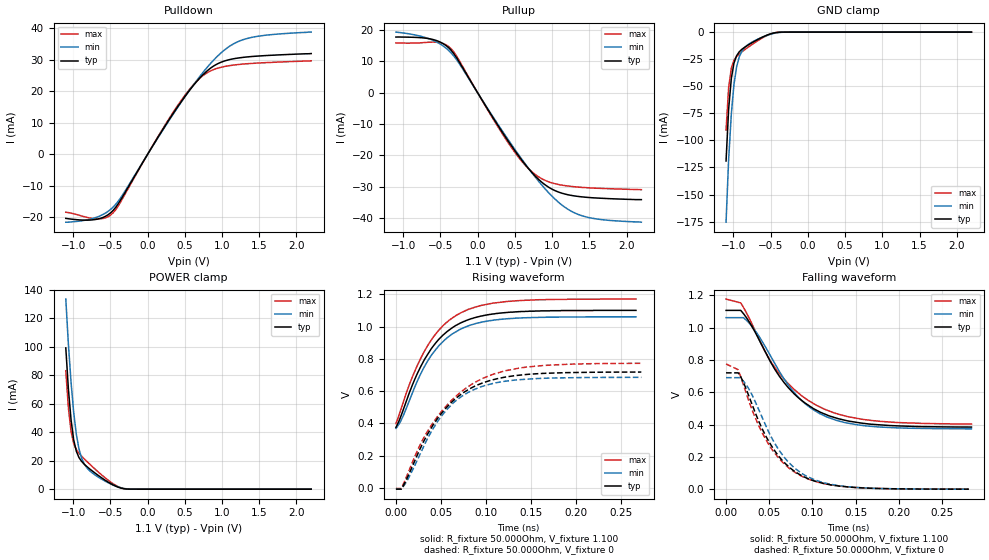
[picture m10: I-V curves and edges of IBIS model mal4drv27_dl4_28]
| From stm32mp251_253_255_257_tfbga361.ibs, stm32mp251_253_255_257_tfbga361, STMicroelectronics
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[Model] mal4drv27_dl4_28
Model_type   I/O
Polarity   Non-Inverting
Enable   Active-High
C_comp   1.656pF   1.654pF   1.662pF
C_comp_pullup   832.475fF   825.290fF   839.619fF
C_comp_pulldown 737.556fF   736.745fF   750.731fF
Vinh = 413.000mV
Vinl = 293.000mV
Vmeas = 353.000mV
Vref = 0.00V
Rref = 50Ohms
Cref = 0pF
[Model Spec]
Vinh   413.000mV   400.000mV   435.000mV
Vinl   293.000mV   280.000mV   315.000mV
Vmeas   353.000mV   340.000mV   375.000mV
Vref   0.00V   0.00V   0.00V
D_overshoot_ampl_h 0.3 NA   NA
D_overshoot_ampl_l 0.3 NA   NA
D_overshoot_area_l 100.000m NA   NA
D_overshoot_area_h 100.000m NA   NA
[Receiver Thresholds]
Vth = 353.000mV
Vth_min = 340.000mV
Vth_max = 375.000mV
Vinh_ac = 600.000mV
Vinh_dc = 600.000mV
Vinl_ac = -600.000mV
Vinl_dc = -600.000mV
Tslew_ac = 5.000ns
Threshold_sensitivity = 0.5
Reference_supply Pullup_ref
[Temperature Range]   25.000   125.000   -40.000
[Voltage Range]   1.100V   1.060V   1.170V
[GND Clamp Reference]   0.00V   0.00V   0.00V
[C Comp Corner]
| variable   typ   min   max
C_comp 1.662pF   1.656pF   1.654pF
C_comp_pullup 832.475fF   839.619fF   825.290fF
C_comp_pulldown 736.745fF   750.731fF   737.556fF
[Pulldown Reference]   0.00V   0.00V   0.00V
[POWER Clamp Reference]   1.100V   1.060V   1.170V
[Pullup Reference]   1.100V   1.060V   1.170V
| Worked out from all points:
|   slope of the pulldown table from 0 to 0.165 V, typ, clamps not added: 25.9 ohm
|   slope of the pullup table from 0 to 0.165 V, typ, clamps not added: 25.9 ohm
|   GND clamp passes 1 mA (typ) near -0.47 V on its own axis
|   POWER clamp passes 1 mA (typ) near -0.37 V on its own axis
|   rising waveform, R_fixture 50.000Ohm, V_fixture 1.100: 20-80 % time 43.6ps typ, 42.6ps min, 45ps max; typ from 0.376 V to 1.1 V
|   rising waveform, R_fixture 50.000Ohm, V_fixture 0: 20-80 % time 52.1ps typ, 47.8ps min, 59.7ps max; typ from -0.007 V to 0.718 V
|   falling waveform, R_fixture 50.000Ohm, V_fixture 1.100: 20-80 % time 58ps typ, 55.1ps min, 62.7ps max; typ from 1.11 V to 0.384 V
|   falling waveform, R_fixture 50.000Ohm, V_fixture 0: 20-80 % time 45.1ps typ, 44.8ps min, 46ps max; typ from 0.72 V to 0 V
[GND Clamp]
-1.099V   -119mA     -175.5mA   -90.46mA
-1.064V   -70.81mA   -117.3mA   -51.1mA
-1.028V   -42.76mA   -75.52mA   -33.21mA
-992.7mV  -28.64mA   -48.36mA   -25.94mA
-957.3mV  -21.83mA   -32.18mA   -22.47mA
-921.8mV  -18.22mA   -22.95mA   -20.16mA
-886.4mV  -15.9mA    -17.64mA   -18.21mA
-815.5mV  -12.5mA    -12.17mA   -14.62mA
-567.3mV  -3.324mA   -3.512mA   -3.774mA
-460.9mV  -879.1uA   -1.269mA   -863.6uA
-390mV    -181.5uA   -432.7uA   -123.2uA
2.198V    31.48nA    451.7nA    3.508nA
[Power Clamp]
-1.098V   99.1mA     133.3mA    83.09mA
-1.063V   70.06mA    101.6mA    56.85mA
-1.027V   48.48mA    74.82mA    40.4mA
-991.8mV  34.54mA    53.74mA    31.95mA
-956.4mV  26.58mA    38.45mA    27.74mA
-920.9mV  22.17mA    28.22mA    25.15mA
-885.5mV  19.46mA    21.74mA    23.1mA
-814.5mV  15.82mA    14.94mA    19.43mA
-743.6mV  12.83mA    11.41mA    15.93mA
-460mV    2.904mA    2.84mA     3.733mA
-282.7mV  117.7uA    274uA      108uA
2.199V    -10.68nA   -391.6nA   -2.283nA
[Pulldown]
-1.099V   -20.3mA    -21.5mA    -18.34mA
-673.6mV  -20.53mA   -19.84mA   -20.47mA
-567.3mV  -19.66mA   -18.64mA   -20.13mA
-460.9mV  -17.71mA   -16.66mA   -18.48mA
-319.1mV  -12.76mA   -12.24mA   -13.29mA
106.4mV   4.13mA     4.019mA    4.282mA
425.4mV   15.78mA    15.6mA     16.18mA
673.6mV   23.44mA    23.8mA     23.48mA
886.4mV   27.95mA    29.81mA    26.82mA
1.099V    29.98mA    34.19mA    28.07mA
1.312V    30.77mA    36.51mA    28.63mA
2.198V    31.9mA     38.7mA     29.59mA
[Pullup]
-1.098V   17.8mA     19.39mA    15.94mA
-601.8mV  17.02mA    16.78mA    16.19mA
-460mV    15.66mA    14.9mA     15.68mA
-353.6mV  13.5mA     12.65mA    13.99mA
-282.7mV  11.19mA    10.55mA    11.72mA
249.1mV   -9.546mA   -9.223mA   -9.941mA
497.3mV   -18.38mA   -17.98mA   -18.91mA
710mV     -24.94mA   -24.94mA   -24.83mA
958.2mV   -30.21mA   -32.01mA   -28.45mA
1.206V    -32.51mA   -37.08mA   -29.74mA
1.419V    -33.26mA   -39.37mA   -30.22mA
2.199V    -34.1mA    -41.3mA    -30.92mA
[Ramp]
R_load=50.000Ohm
dV/dt_r   430.530mV/49.500ps  411.899mV/46.500ps  462.390mV/53.500ps
dV/dt_f   430.530mV/52.500ps  411.899mV/51.000ps  462.390mV/55.500ps
[Rising waveform]
R_fixture=50.000Ohm
V_fixture=1.100
V_fixture_min=1.060
V_fixture_max=1.170
0s        376.3mV    369.6mV    399.1mV
8ps       482.4mV    445.6mV    530.3mV
19ps      647.6mV    599.2mV    697.8mV
35ps      825.4mV    784mV      879.1mV
44ps      897mV      855.2mV    952.6mV
54ps      954.9mV    916.5mV    1.014V
74ps      1.027V     989mV      1.09V
95ps      1.065V     1.027V     1.131V
125ps     1.088V     1.049V     1.156V
267ps     1.1V       1.06V      1.17V
[Rising waveform]
R_fixture=50.000Ohm
V_fixture=0
0s        -6.743mV   -6.219mV   -2.378mV
6ps       -6.743mV   -6.219mV   -2.378mV
10ps      32.97mV    23.66mV    46.56mV
29ps      268.2mV    236.9mV    290.9mV
50ps      458.2mV    441.2mV    469.7mV
72ps      578.7mV    563.4mV    593.7mV
95ps      648.1mV    627.6mV    674.9mV
121ps     686.5mV    661.1mV    725.5mV
149ps     704.9mV    675.9mV    751.2mV
273ps     718.2mV    685.4mV    772.3mV
[Falling waveform]
R_fixture=50.000Ohm
V_fixture=1.100
V_fixture_min=1.060
V_fixture_max=1.170
0s        1.106V     1.061V     1.176V
17ps      1.106V     1.061V     1.152V
26ps      1.042V     1.032V     1.066V
44ps      863.1mV    894.4mV    863.4mV
58ps      728.5mV    762mV      740.6mV
80ps      583.5mV    590mV      611.6mV
104ps     490.3mV    481.5mV    520.7mV
126ps     442mV      428.3mV    470.2mV
162ps     405.2mV    391.4mV    429.2mV
284ps     384.3mV    373.3mV    403mV
[Falling waveform]
R_fixture=50.000Ohm
V_fixture=0
0s        719.6mV    689.8mV    774.7mV
14ps      719.6mV    689.8mV    739.1mV
22ps      637.2mV    656mV      614.5mV
35ps      456.6mV    526.3mV    426.9mV
49ps      299.2mV    357.7mV    280.3mV
66ps      172.9mV    205.9mV    163.1mV
84ps      94.33mV    111.8mV    90.04mV
107ps     43.45mV    49.57mV    42.11mV
137ps     15.62mV    17.23mV    16.07mV
281ps     141.4uV    164.3uV    160.5uV
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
